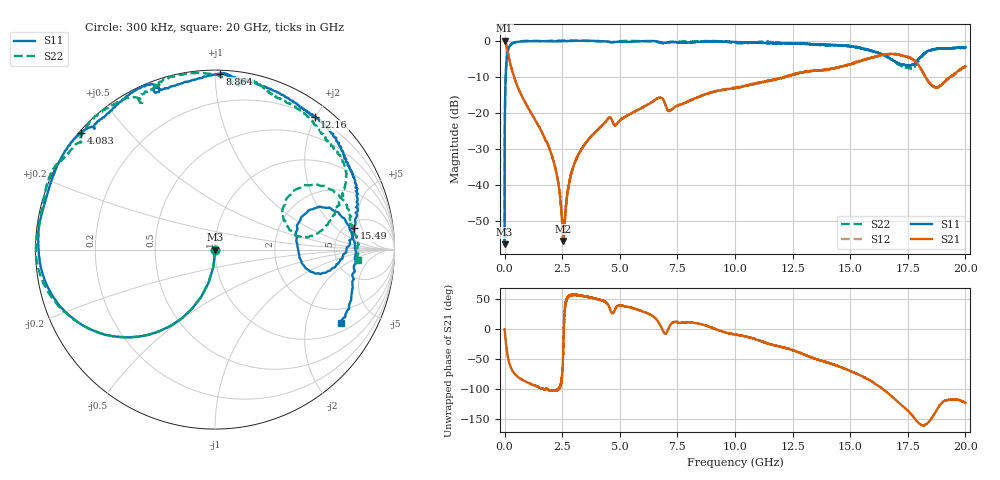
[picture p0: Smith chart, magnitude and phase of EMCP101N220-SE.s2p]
!EMCP101N220
!Johanson Technology Inc.
!www.johansontechnology.com
!Test Board Conditions:
!Substrate Type  RO4350B
!Substrate Thickness  10 mil
!Substrate Dk  3.66
!TL Type: GCPW
!TL Trace Width  20 mil
!TL Gap  10 mil
!PART MODE SINGLE ENDED (AKA BYPASS)
!DUT TOPOLOGY	SERIES-SHUNT
# MHz S  dB  R 50
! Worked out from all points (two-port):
!   20001 points, 300 kHz to 20 GHz, reference 50 ohm
!   highest |S21| = 0.00 dB at 1.3 MHz (marker M1); lowest = -55.4 dB at 2.553 GHz (marker M2)
!   |S21| within 3 dB of the highest: start of sweep to 135.1 MHz
!   lowest |S11| = -56.3 dB at 300 kHz (marker M3), VSWR 1.00, Z = 50.1 - j0.121 ohm
!   |S11| at or under -10 dB: start of sweep to 45.96 MHz
!   |S22| runs from -56.8 to 0.1 dB; largest |S21 - S12| = 0.021
!   S11 on the Smith chart (normalised r, x): 300 kHz: 1.00, -0.00; 4.083 GHz: 0.01, +0.37; 8.864 GHz: 0.02, +1.03; 12.16 GHz: 0.20, +1.99; 15.49 GHz: 5.89, +3.68; 20 GHz: 1.29, -3.20
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0.3  -56.31 -52.5  -0.02 -0.2  -0.00 -0.2  -56.85 -43.7
1.3  -40.66 -88.0  -0.00 -0.6  -0.01 -0.6  -40.59 -88.6
104.298  -4.39 -128.0  -2.02 -37.7  -2.00 -37.7  -4.43 -127.9
226.297  -1.41 -150.4  -5.80 -59.6  -5.78 -59.6  -1.43 -150.1
678.29  -0.23 -173.9  -14.35 -82.3  -14.36 -82.5  -0.13 -172.1
2015.27  -0.14 166.0  -31.09 -102.2  -31.04 -102.3  -0.05 163.4
2553.262  -0.11 158.2  -55.44 -23.8  -55.18 -25.2  0.05 157.1
2869.257  -0.05 153.5  -37.32 57.0  -37.39 56.1  0.07 154.7
3334.25  -0.01 147.1  -30.03 56.0  -30.03 55.9  0.01 151.8
4083.239  -0.09 139.0  -24.34 49.6  -24.36 49.7  -0.18 146.9
6667.2  -0.25 109.5  -15.84 12.3  -15.81 11.8  -0.42 117.3
7168.192  -0.32 110.7  -19.37 5.5  -19.39 5.3  -0.43 115.7
8864.167  -0.18 88.3  -14.50 4.4  -14.54 4.3  -0.07 103.9
10000.15  -0.37 82.5  -13.11 -9.0  -12.92 -8.8  -0.58 83.0
12163.12  -0.68 53.1  -10.07 -31.0  -9.90 -30.7  -0.69 69.8
13334.1  -0.95 37.9  -8.38 -47.3  -8.35 -47.8  -1.00 51.1
15488.07  -2.12 8.9  -5.56 -77.9  -5.39 -78.3  -2.04 25.0
16667.05  -4.67 -13.0  -3.68 -107.5  -3.81 -106.6  -4.64 9.2
17678.03  -6.70 12.0  -5.02 -143.0  -4.91 -142.3  -7.51 25.6
18188.03  -3.57 20.6  -9.16 -160.4  -8.98 -160.5  -3.88 34.1
18791.02  -2.16 3.4  -12.86 -132.5  -12.82 -133.6  -2.27 19.7
20000  -1.76 -30.4  -7.14 -122.8  -7.23 -120.4  -1.95 -4.3
